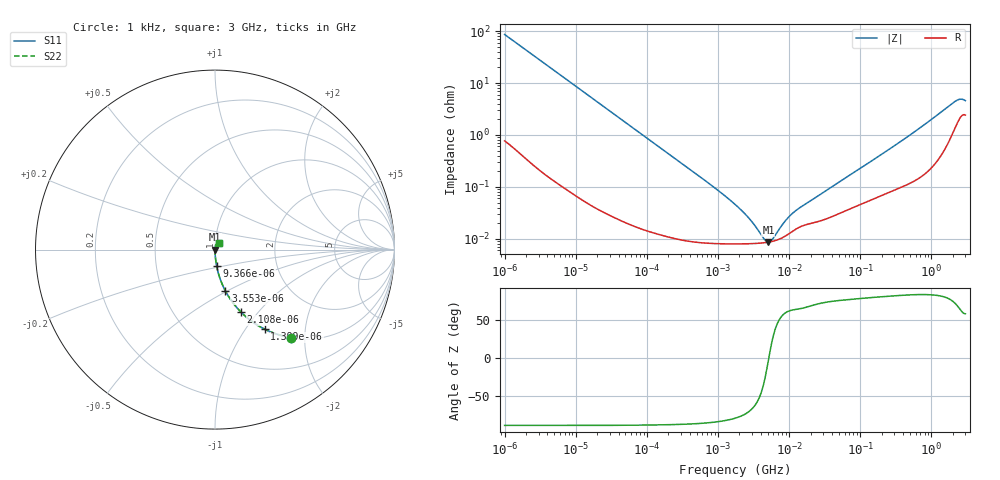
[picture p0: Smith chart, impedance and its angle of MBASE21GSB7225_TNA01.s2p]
! MBASE21GSB7225_TNA01  S-PARAMETER MODEL  ( Standard Model )
! Model Generated by TAIYO YUDEN Corporation (http://www.ty-top.com)
! Version 1.0
! TAIYO YUDEN Control No. 220601
! Copyright(c) 2012 TAIYO YUDEN CO.,LTD. All Rights Reserved.
! Product Description (link to TY-COMPAS)
! https://ds.yuden.co.jp/TYCOMPAS/or/detail?pn=MBASE21GSB7225KTNA01&u=M
! Products Name : Multilayer Ceramic Capacitors
! Characteristics :
!  Capacitance : 2.2 [uF] , Rated Voltage : 16 [V] , TCC : X7R
!  Case Size : 2.0 x 1.25 / 0.079 x 0.049 [mm/inch] , Thickness : 1.25 / 0.049 [mm/inch]
!  (Conditions: Temperature = 25 [degC] , DC Bias Voltage = 0 [V])
! External Node Assignments :
!  1  o---| |---o  2
! GND o---------o GND
! Frequency Range : 1kHz  -  3GHz  [ 401 STEP ]
# MHZ S RI R 50
! Freq[MHz].  S11 Real  S11 Imag  S21 Real  S21 Imag  S12 Real  S12 Imag  S22 Real  S22 Imag
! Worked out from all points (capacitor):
!   401 points, 1 kHz to 3 GHz, reference 50 ohm
!   read as one part in series: C = 1.85 uF near 1.077 kHz
!   lowest |Z| = 8.67 mohm at 5.107 MHz (marker M1)
!   series resonance near 5.182 MHz, so ESL is about 510 pH
!   S11 on the Smith chart (normalised r, x): 1 kHz: 1.02, -1.72; 1.399 kHz: 1.01, -1.23; 2.108 kHz: 1.01, -0.82; 3.553 kHz: 1.00, -0.49; 9.366 kHz: 1.00, -0.19; 3 GHz: 1.05, +0.08
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0.001  0.4258 -0.49  0.5742 0.49  0.5742 0.49  0.4258 -0.49
0.001399  0.2769 -0.4432  0.7231 0.4432  0.7231 0.4432  0.2769 -0.4432
0.002108  0.1458 -0.3489  0.8542 0.3489  0.8542 0.3489  0.1458 -0.3489
0.003553  0.0576 -0.2293  0.9424 0.2293  0.9424 0.2293  0.0576 -0.2293
0.009366  0.00924 -0.0919  0.9908 0.0919  0.9908 0.0919  0.00924 -0.0919
0.01216  0.00565 -0.0711  0.9943 0.0711  0.9943 0.0711  0.00565 -0.0711
0.033275  0.000953 -0.0262  0.999 0.0262  0.999 0.0262  0.000953 -0.0262
0.147855  0.000157 -0.00595  0.9998 0.00595  0.9998 0.00595  0.000157 -0.00595
0.762639  8.33e-05 -0.00114  0.9999 0.00114  0.9999 0.00114  8.33e-05 -0.00114
1.732051  8.02e-05 -0.000455  0.9999 0.000455  0.9999 0.000455  8.02e-05 -0.000455
2.812335  8.08e-05 -0.000223  0.9999 0.000223  0.9999 0.000223  8.08e-05 -0.000223
4.238263  8.37e-05 -6.98e-05  0.9999 6.98e-05  0.9999 6.98e-05  8.37e-05 -6.98e-05
5.106836  8.65e-05 -4.97e-06  0.9999 4.97e-06  0.9999 4.97e-06  8.65e-05 -4.97e-06
5.711239  8.92e-05 3.38e-05  0.9999 -3.38e-05  0.9999 -3.38e-05  8.92e-05 3.38e-05
6.153411  9.15e-05 5.99e-05  0.9999 -5.99e-05  0.9999 -5.99e-05  9.15e-05 5.99e-05
8.606987  0.000111 0.000182  0.9999 -0.000182  0.9999 -0.000182  0.000111 0.000182
11.1738  0.00014 0.000278  0.9999 -0.000278  0.9999 -0.000278  0.00014 0.000278
21.06097  0.000202 0.000529  0.9998 -0.000529  0.9998 -0.000529  0.000202 0.000529
256.0921  0.000816 0.00527  0.9992 -0.00527  0.9992 -0.00527  0.000816 0.00527
2066.299  0.0136 0.04  0.9864 -0.04  0.9864 -0.04  0.0136 0.04
2489.759  0.0221 0.0422  0.9779 -0.0422  0.9779 -0.0422  0.0221 0.0422
3000  0.025 0.0371  0.975 -0.0371  0.975 -0.0371  0.025 0.0371
